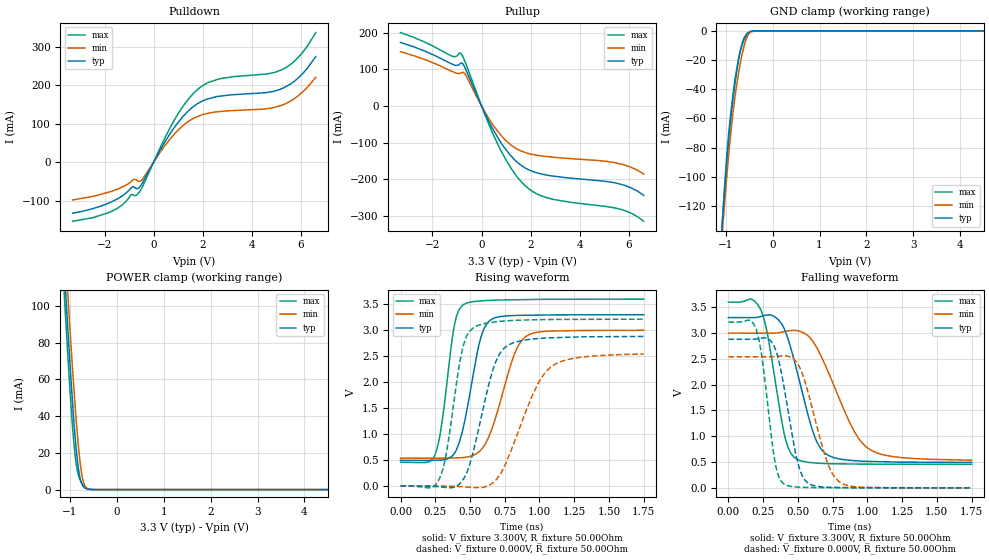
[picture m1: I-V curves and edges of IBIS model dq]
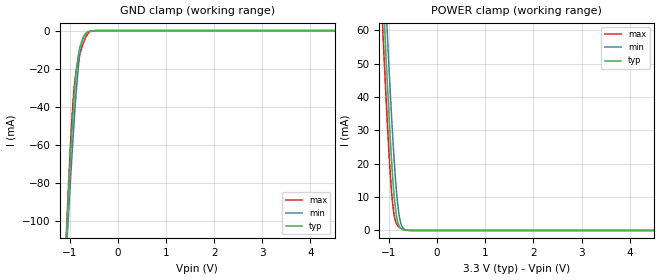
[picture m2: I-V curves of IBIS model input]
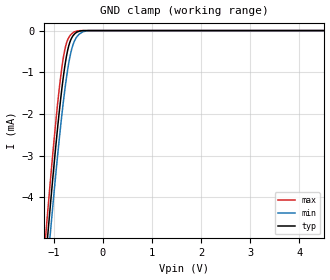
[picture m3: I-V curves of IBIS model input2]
| y27b.ibs * IBIS 3.2 Model
| 512Mb SDRAM
[IBIS Ver]   3.2
[File name]   y27b_die.ibs
[File rev]   2.4
[Date]   04/14/2004
[Source]   From silicon level SPICE model at Micron Technology, Inc.
   Micron Technology, Inc.
   8000 S. Federal Way
   P.O. Box 6 M/S: 1-711
   Boise ID 83707-0006
[Notes]   Rev 1.0: 05/15/2003
   - initial file creation
   Rev 2.0: 06/17/2003
   - Matched the I-V curves of the dq models
   to silicon measurements
   Rev 2.1: 07/17/2003
   - DQ model V-T curves updated due to spice model change
   to match c_comp in slow and fast corner cases.
   Rev 2.2: 10/16/2003
   - added complete pin parasitics for the x16 54-ball FBGA
   Rev 2.3: 04/07/2004
   - updated C_comp values for all models
   - matched I-V curves to latest silicon measurements
   - removed FBGA packages - not supported
   Rev 2.4: 04/14/2004
   - updated DQ model due to circuit change
   - all models updated for 40C typical temperature
   Rev TL1.0 created die only model  Teraspeed Labs
[Disclaimer]  This software code and all associated documentation, comments
   or other information (collectively "Software") is provided
   "AS IS" without warranty of any kind. MICRON TECHNOLOGY, INC.
   ("MTI") EXPRESSLY DISCLAIMS ALL WARRANTIES EXPRESS OR IMPLIED,
   INCLUDING BUT NOT LIMITED TO, NONINFRINGEMENT OF THIRD PARTY
   RIGHTS, AND ANY IMPLIED WARRANTIES OF MERCHANTABILITY OR
   FITNESS FOR ANY PARTICULAR PURPOSE. MTI DOES NOT WARRANT THAT
   THE SOFTWARE WILL MEET YOUR REQUIREMENTS, OR THAT THE
   OPERATION OF THE SOFTWARE WILL BE UNINTERRUPTED OR ERROR-FREE.
   FURTHERMORE, MTI DOES NOT MAKE ANY REPRESENTATIONS REGARDING
   THE USE OR THE RESULTS OF THE USE OF THE SOFTWARE IN TERMS OF
   ITS CORRECTNESS, ACCURACY, RELIABILITY, OR OTHERWISE. THE
   ENTIRE RISK ARISING OUT OF USE OR PERFORMANCE OF THE SOFTWARE
   REMAINS WITH YOU. IN NO EVENT SHALL MTI, ITS AFFILIATED
   COMPANIES OR THEIR SUPPLIERS BE LIABLE FOR ANY DIRECT,
   INDIRECT, CONSEQUENTIAL, INCIDENTAL, OR SPECIAL DAMAGES
   (INCLUDING, WITHOUT LIMITATION, DAMAGES FOR LOSS OF PROFITS,
   BUSINESS INTERRUPTION, OR LOSS OF INFORMATION) ARISING OUT OF
   YOUR USE OF OR INABILITY TO USE THE SOFTWARE, EVEN IF MTI HAS
   BEEN ADVISED OF THE POSSIBILITY OF SUCH DAMAGES. Because some
   jurisdictions prohibit the exclusion or limitation of
   liability for consequential or incidental damages, the above
   limitation may not apply to you.
[Copyright]   Copyright 2003 Micron Technology, Inc. All rights reserved.
|   COMPONENT: Y27B SDRAM
[Component]   Y27B
[Manufacturer]   Micron Technology, Inc.
[Package]   | Die
|variable   typ   min   max
R_pkg   0.0000   0.0000   0.0000
L_pkg   0.0000   0.0000   0.0000
C_pkg   0.0000   0.0000   0.0000
[Pin]  signal_name   model_name  R_pin   L_pin   C_pin
1   DNU   NC
2   DNU   NC
3   VSS   GND
4   VDD   POWER
5   DQ7   dq
6   DQ0   dq
7   VSSQ   GND
8   VDDQ   POWER
9   DNU   NC
10   DNU   NC
11   DQ6   dq
12   DQ1   dq
13   VDDQ   POWER
14   VSSQ   GND
15   DNU   NC
16   DNU   NC
17   DQ5   dq
18   DQ2   dq
19   VSSQ   GND
20   VDDQ   POWER
21   DNU   NC
22   DNU   NC
23   DQ4   dq
24   DQ3   dq
25   VDDQ   POWER
26   VSSQ   GND
27   DNU   NC
28   DNU   NC
29   DNU   NC
30   DNU   NC
31   DNU   NC
32   DNU   NC
33   VSS   GND
34   VDD   POWER
35   VSS   GND
36   VDD   POWER
37   DNU   NC
38   DQM   input
39   DNU   NC
40   DNU   NC
41   WE#   input
42   DNU   NC
43   CAS#   input
44   CLK   clk
45   RAS#   input
46   CKE   input
47   CS#   input
48   A12   input2
49   BA0   input
50   A11   input
51   BA1   input
52   A9   input
53   A10/AP  input
54   A8   input
55   A0   input
56   A7   input
57   A1   input
58   A6   input
59   A2   input
60   A5   input
61   A3   input
62   A4   input
63   VDD   POWER
64   VSS   GND
65   NC   NC
66   NC   NC
| Models and submodels in the file (4): dq (I/O), input (Input), input2 (Input), clk (Input)
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|   dq MODEL
[Model]   dq
Model_type   I/O
Vinl = 800.000mV
Vinh = 2.000V
Vmeas = 1.500V
Cref = 50.000pF
|   typ   min   max
C_comp   3.940pF   3.670pF   4.270pF
[Voltage Range]   3.300V   3.000V   3.600V
| Junction Temperature (Ambient temp is 25C typ, 70C min, 0C max)
[Temperature Range]   40.0   85.0   0.0
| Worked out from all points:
|   slope of the pulldown table from 0 to 0.495 V, typ, clamps not added: 8.81 ohm
|   slope of the pullup table from 0 to 0.495 V, typ, clamps not added: 7.4 ohm
|   GND clamp passes 1 mA (typ) near -0.51 V on its own axis
|   POWER clamp passes 1 mA (typ) near -0.68 V on its own axis
|   falling waveform, V_fixture 3.300V, R_fixture 50.00Ohm: 20-80 % time 167ps typ, 245ps min, 117ps max; typ from 3.3 V to 0.494 V
|   rising waveform, V_fixture 3.300V, R_fixture 50.00Ohm: 20-80 % time 121ps typ, 167ps min, 89.1ps max; typ from 0.494 V to 3.3 V
|   rising waveform, V_fixture 0.000V, R_fixture 50.00Ohm: 20-80 % time 158ps typ, 234ps min, 110ps max; typ from 0 V to 2.88 V
|   falling waveform, V_fixture 0.000V, R_fixture 50.00Ohm: 20-80 % time 116ps typ, 156ps min, 87.7ps max; typ from 2.88 V to 0 V
[Pulldown]
|   Voltage   I(typ)   I(min)   I(max)
-3.3V     -133mA     -98.6mA    -153.9mA
-1.75V    -104.5mA   NA         NA
-870mV    -64.04mA   NA         NA
-690mV    -69.24mA   NA         -85.9mA
-470mV    -55.81mA   NA         NA
930mV     97.73mA    NA         NA
1.35V     129.2mA    NA         NA
1.94V     157.4mA    NA         NA
2.58V     170.3mA    NA         NA
5.2V      190.1mA    NA         NA
5.91V     219.9mA    NA         NA
6.6V      274.2mA    220.3mA    336.5mA
[GND Clamp]
|   Voltage   I(typ)   I(min)   I(max)
-3.3V     -1.416A    -1.252A    -1.676A
-1.07V    -130.7mA   -137.9mA   NA
-1.04V    -116.8mA   -125.3mA   -114.7mA
-990mV    -95.11mA   NA         NA
-950mV    -79.52mA   NA         NA
-890mV    -59.55mA   -69.81mA   NA
-810mV    -38.13mA   NA         NA
-730mV    -20.83mA   NA         NA
-670mV    -11.11mA   NA         -11.77mA
-570mV    -2.721mA   NA         NA
-490mV    -620.9uA   NA         NA
6.6V      0A         0A         0A
[Pullup]
|   Voltage   I(typ)   I(min)   I(max)
-3.3V     173.9mA    148.7mA    200.8mA
-1.27V    116.6mA    NA         NA
-990mV    111mA      NA         NA
-840mV    117.4mA    NA         143.8mA
-650mV    100.9mA    NA         NA
230mV     -32.9mA    NA         NA
810mV     -102mA     NA         NA
1.36V     -147.8mA   NA         NA
2V        -176.6mA   NA         -229.9mA
2.76V     -189.9mA   NA         NA
5.54V     -211.3mA   NA         NA
6.6V      -243.9mA   -185.4mA   -314.8mA
[POWER Clamp]
|   Voltage   I(typ)   I(min)   I(max)
-3.3V     1.22A      1.202A     1.244A
-1.13V    125.4mA    NA         NA
-1.08V    103.5mA    NA         NA
-1.05V    90.59mA    109.2mA    NA
-1.01V    73.93mA    NA         59.49mA
-950mV    50.38mA    NA         36.91mA
-870mV    23.7mA     NA         NA
-810mV    10.11mA    NA         NA
-770mV    5.039mA    NA         NA
-730mV    2.385mA    NA         NA
-670mV    702.4uA    1.675mA    NA
6.6V      0A         0A         0A
[Ramp]
R_load = 50.00Ohm
|   typ   min   max
dV/dt_r   1.729V/158.003ps   1.525V/233.558ps   1.928V/109.916ps
dV/dt_f   1.684V/166.713ps   1.479V/244.893ps   1.886V/117.427ps
[Falling Waveform]
V_fixture = 3.300V
V_fixture_min = 3.000V
V_fixture_max = 3.600V
R_fixture = 50.00Ohm
|   Time   V(typ)   V(min)   V(max)
0s        3.3V       3V         3.6V
220ps     3.312V     NA         NA
270ps     3.351V     NA         NA
380ps     3.192V     NA         NA
420ps     2.959V     NA         NA
480ps     2.402V     NA         NA
620ps     996.2mV    NA         NA
720ps     627.2mV    NA         NA
970ps     515.8mV    NA         NA
1.75ns    493.6mV    535.2mV    456.5mV
[Rising Waveform]
V_fixture = 3.300V
V_fixture_min = 3.000V
V_fixture_max = 3.600V
R_fixture = 50.00Ohm
|   Time   V(typ)   V(min)   V(max)
0s        493.6mV    535.2mV    456.5mV
210ps     492mV      NA         NA
300ps     499.5mV    NA         NA
390ps     637.3mV    NA         NA
450ps     1.106V     NA         NA
570ps     2.78V      NA         NA
660ps     3.218V     NA         NA
850ps     3.287V     NA         NA
1.14ns    3.297V     NA         NA
1.75ns    3.3V       3V         3.6V
[Rising Waveform]
V_fixture = 0.000V
V_fixture_min = 0.000V
V_fixture_max = 0.000V
R_fixture = 50.00Ohm
|   Time   V(typ)   V(min)   V(max)
0s        4.443uV    -198.5nV   4.058uV
250ps     -10.22mV   NA         NA
350ps     -35.72mV   NA         NA
440ps     82.71mV    NA         NA
530ps     728.7mV    NA         NA
670ps     2.279V     NA         NA
780ps     2.722V     NA         NA
1.04ns    2.851V     NA         NA
1.3ns     2.873V     NA         NA
1.75ns    2.881V     2.542V     3.214V
[Falling Waveform]
V_fixture = 0.000V
V_fixture_min = 0.000V
V_fixture_max = 0.000V
R_fixture = 50.00Ohm
|   Time   V(typ)   V(min)   V(max)
0s        2.881V     2.542V     3.214V
200ps     2.886V     NA         NA
240ps     2.903V     NA         NA
330ps     2.742V     NA         NA
400ps     1.957V     NA         NA
500ps     479.3mV    NA         NA
580ps     79.6mV     NA         NA
740ps     9.224mV    NA         NA
1.06ns    1.366mV    NA         NA
1.75ns    4.443uV    -198.5nV   4.058uV
|   input MODEL
[Model]   input
Model_type   Input
Vinl = 800.000mV
Vinh = 2.000V
|   typ   min   max
C_comp   2.130pF   1.940pF   2.370pF
[Voltage Range]   3.300V   3.000V   3.600V
| Junction Temperature (Ambient temp is 25C typ, 70C min, 0C max)
[Temperature Range]   40.0   85.0   0.0
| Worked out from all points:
|   GND clamp passes 1 mA (typ) near -0.64 V on its own axis
|   POWER clamp passes 1 mA (typ) near -0.77 V on its own axis
[GND Clamp]
|   Voltage   I(typ)   I(min)   I(max)
-3.3V     -1.431A    -1.275A    -1.646A
-1.07V    -109mA     -116.8mA   -106mA
-1.05V    -98.79mA   -107.6mA   -94.47mA
-990mV    -69.48mA   -80.79mA   -62.28mA
-950mV    -51.55mA   -63.83mA   -44.07mA
-910mV    -35.7mA    -47.9mA    -30.18mA
-850mV    -18.03mA   -27.05mA   -18.55mA
-790mV    -8.784mA   -12.06mA   -12.42mA
-750mV    -5.487mA   -6.201mA   -9.085mA
-690mV    -2.425mA   -2.143mA   -4.761mA
-610mV    -575.3uA   -540.4uA   -1.197mA
6.6V      0A         0A         0A
[POWER Clamp]
|   Voltage   I(typ)   I(min)   I(max)
-3.3V     840.5mA    849.5mA    834.5mA
-1.13V    73.22mA    88.26mA    60.66mA
-1.09V    60.82mA    75.77mA    48.38mA
-1.05V    48.83mA    63.59mA    36.68mA
-1.03V    43.05mA    57.65mA    31.13mA
-950mV    21.99mA    35.23mA    12.36mA
-910mV    13.47mA    25.22mA    6.325mA
-870mV    7.092mA    16.47mA    3.065mA
-830mV    3.228mA    9.474mA    1.654mA
-790mV    1.387mA    4.671mA    1.002mA
-710mV    274.6uA    773.7uA    NA
6.6V      0A         0A         0A
|   input2 MODEL
[Model]   input2
Model_type   Input
| Used for A12. Contains no Power Clamp structures
Vinl = 800.000mV
Vinh = 2.000V
|   typ   min   max
C_comp   2.130pF   1.940pF   2.370pF
[Voltage Range]   3.300V   3.000V   3.600V
| Junction Temperature (Ambient temp is 25C typ, 70C min, 0C max)
[Temperature Range]   40.0   85.0   0.0
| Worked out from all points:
|   GND clamp passes 1 mA (typ) near -0.79 V on its own axis
[GND Clamp]
|   Voltage   I(typ)   I(min)   I(max)
-3.3V     -38.47mA   -38.51mA   -38.55mA
-1.18V    -5.679mA   -6.32mA    -5.116mA
-1.14V    -5.124mA   NA         -4.552mA
-1.1V     -4.578mA   NA         -3.999mA
-1.06V    -4.044mA   NA         -3.458mA
-920mV    -2.293mA   NA         -1.721mA
-820mV    -1.233mA   -1.85mA    -750.7uA
-760mV    -733.5uA   -1.277mA   -374.2uA
-700mV    -382.1uA   NA         -176.5uA
-570mV    -72.27uA   NA         NA
-380mV    0A         NA         NA
6.6V      0A         0A         0A
[POWER Clamp]
|   Voltage   I(typ)   I(min)   I(max)
-3.3V     0A         0A         0A
0V        0A         0A         0A
6.6V      0A         0A         0A
